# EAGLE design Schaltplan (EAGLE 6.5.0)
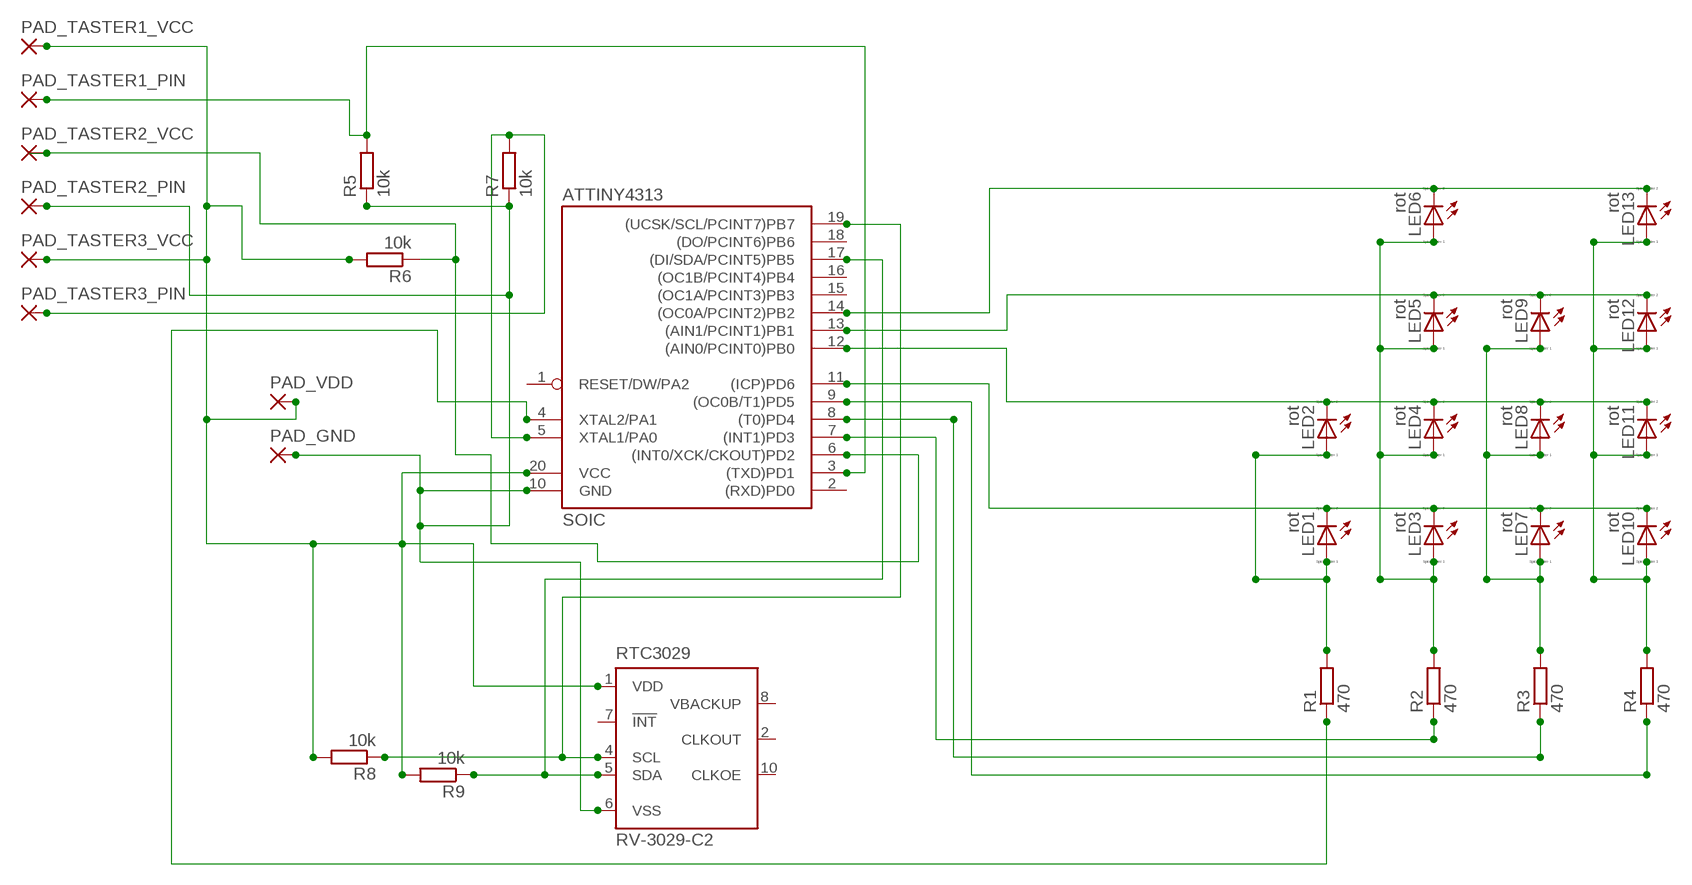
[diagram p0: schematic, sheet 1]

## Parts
ATTINY4313  SOIC  TINY2313P_THM'SOIC'  [SOIC20S]
LED1  rot  LED_ESML0603  [LED_SML0603]
LED2  rot  LED_ESML0603  [LED_SML0603]
LED3  rot  LED_ESML0603  [LED_SML0603]
LED4  rot  LED_ESML0603  [LED_SML0603]
LED5  rot  LED_ESML0603  [LED_SML0603]
LED6  rot  LED_ESML0603  [LED_SML0603]
LED7  rot  LED_ESML0603  [LED_SML0603]
LED8  rot  LED_ESML0603  [LED_SML0603]
LED9  rot  LED_ESML0603  [LED_SML0603]
LED10  rot  LED_ESML0603  [LED_SML0603]
LED11  rot  LED_ESML0603  [LED_SML0603]
LED12  rot  LED_ESML0603  [LED_SML0603]
LED13  rot  LED_ESML0603  [LED_SML0603]
PAD_GND  SMD2  [SMD1,27-2,54]
PAD_TASTER1_PIN  SMD2  [SMD1,27-2,54]
PAD_TASTER1_VCC  SMD2  [SMD1,27-2,54]
PAD_TASTER2_PIN  SMD2  [SMD1,27-2,54]
PAD_TASTER2_VCC  SMD2  [SMD1,27-2,54]
PAD_TASTER3_PIN  SMD2  [SMD1,27-2,54]
PAD_TASTER3_VCC  SMD2  [SMD1,27-2,54]
PAD_VDD  SMD2  [SMD1,27-2,54]
R1  470  R-EU_R0603  [R0603]
R2  470  R-EU_R0603  [R0603]
R3  470  R-EU_R0603  [R0603]
R4  470  R-EU_R0603  [R0603]
R5  10k  R-EU_R0603  [R0603]
R6  10k  R-EU_R0603  [R0603]
R7  10k  R-EU_R0603  [R0603]
R8  10k  R-EU_R0603  [R0603]
R9  10k  R-EU_R0603  [R0603]
RTC3029  RV-3029-C2  [SON-10]

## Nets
N$1: LED1.A LED2.A R1.2
N$2: LED3.A LED4.A LED5.A LED6.A R2.2
N$3: LED7.A LED8.A LED9.A R3.2
N$4: LED10.A LED11.A LED12.A LED13.A R4.2
N$5: ATTINY4313.14((OC0A/PCINT2)PB2) LED6.C LED13.C
N$6: ATTINY4313.13((AIN1/PCINT1)PB1) LED5.C LED9.C LED12.C
N$7: ATTINY4313.12((AIN0/PCINT0)PB0) LED2.C LED4.C LED8.C LED11.C
N$8: ATTINY4313.11((ICP)PD6) LED1.C LED3.C LED7.C LED10.C
N$9: ATTINY4313.9((OC0B/T1)PD5) R4.1
N$10: ATTINY4313.19((UCSK/SCL/PCINT7)PB7) R8.1 RTC3029.4(SCL)
N$11: ATTINY4313.17((DI/SDA/PCINT5)PB5) R9.1 RTC3029.5(SDA)
N$12: ATTINY4313.4(XTAL2/PA1) R1.1
N$13: ATTINY4313.3((TXD)PD1) PAD_TASTER1_PIN.1(P) R5.2
N$14: ATTINY4313.5(XTAL1/PA0) PAD_TASTER3_PIN.1(P) R7.2
N$18: ATTINY4313.8((T0)PD4) R3.1
N$19: ATTINY4313.7((INT1)PD3) R2.1
N$20: ATTINY4313.6((INT0/XCK/CKOUT)PD2) PAD_TASTER2_VCC.1(P) R6.1
N$23: ATTINY4313.20(VCC) PAD_TASTER1_VCC.1(P) PAD_TASTER3_VCC.1(P) PAD_VDD.1(P) R6.2 R8.2 R9.2 RTC3029.1(VDD)
N$24: ATTINY4313.10(GND) PAD_GND.1(P) PAD_TASTER2_PIN.1(P) R5.1 R7.1 RTC3029.6(VSS)
Unconnected: ATTINY4313.1(RESET/DW/PA2) ATTINY4313.2((RXD)PD0) ATTINY4313.15((OC1A/PCINT3)PB3) ATTINY4313.16((OC1B/PCINT4)PB4) ATTINY4313.18((DO/PCINT6)PB6) RTC3029.2(CLKOUT) RTC3029.7(!INT) RTC3029.8(VBACKUP) RTC3029.10(CLKOE)

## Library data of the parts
ATTINY4313 = atmel_THM:TINY2313*P_THM: Features Utilizes the AVR® RISC Architecture AVR® High-performance and Low-power RISC Architecture - 120 Powerful Instructions ? Most Single Clock Cycle Execution - 32 x 8 General Purpose Working Registers - Fully Static Operation Data and Non-volatile Program and Data Memories - 2K Bytes of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
LED1-LED13 = eagle-ltspice:LED_E: LED; SPICEMODEL: NONE; SPICEPREFIX: D; SPICETYPE: diode
PAD_GND PAD_TASTER1_PIN PAD_TASTER1_VCC PAD_TASTER2_PIN PAD_TASTER2_VCC PAD_TASTER3_PIN PAD_TASTER3_VCC PAD_VDD = wirepad:SMD2: SMD PAD
R1-R9 = rcl:R-EU_: RESISTOR, European symbol
RTC3029 = crystal:RV-3029-C2: Highly accurate, DTCXO Temperature Compensated Real Time Clock / Calendar Module with I2C Interface. Source: Data shhet

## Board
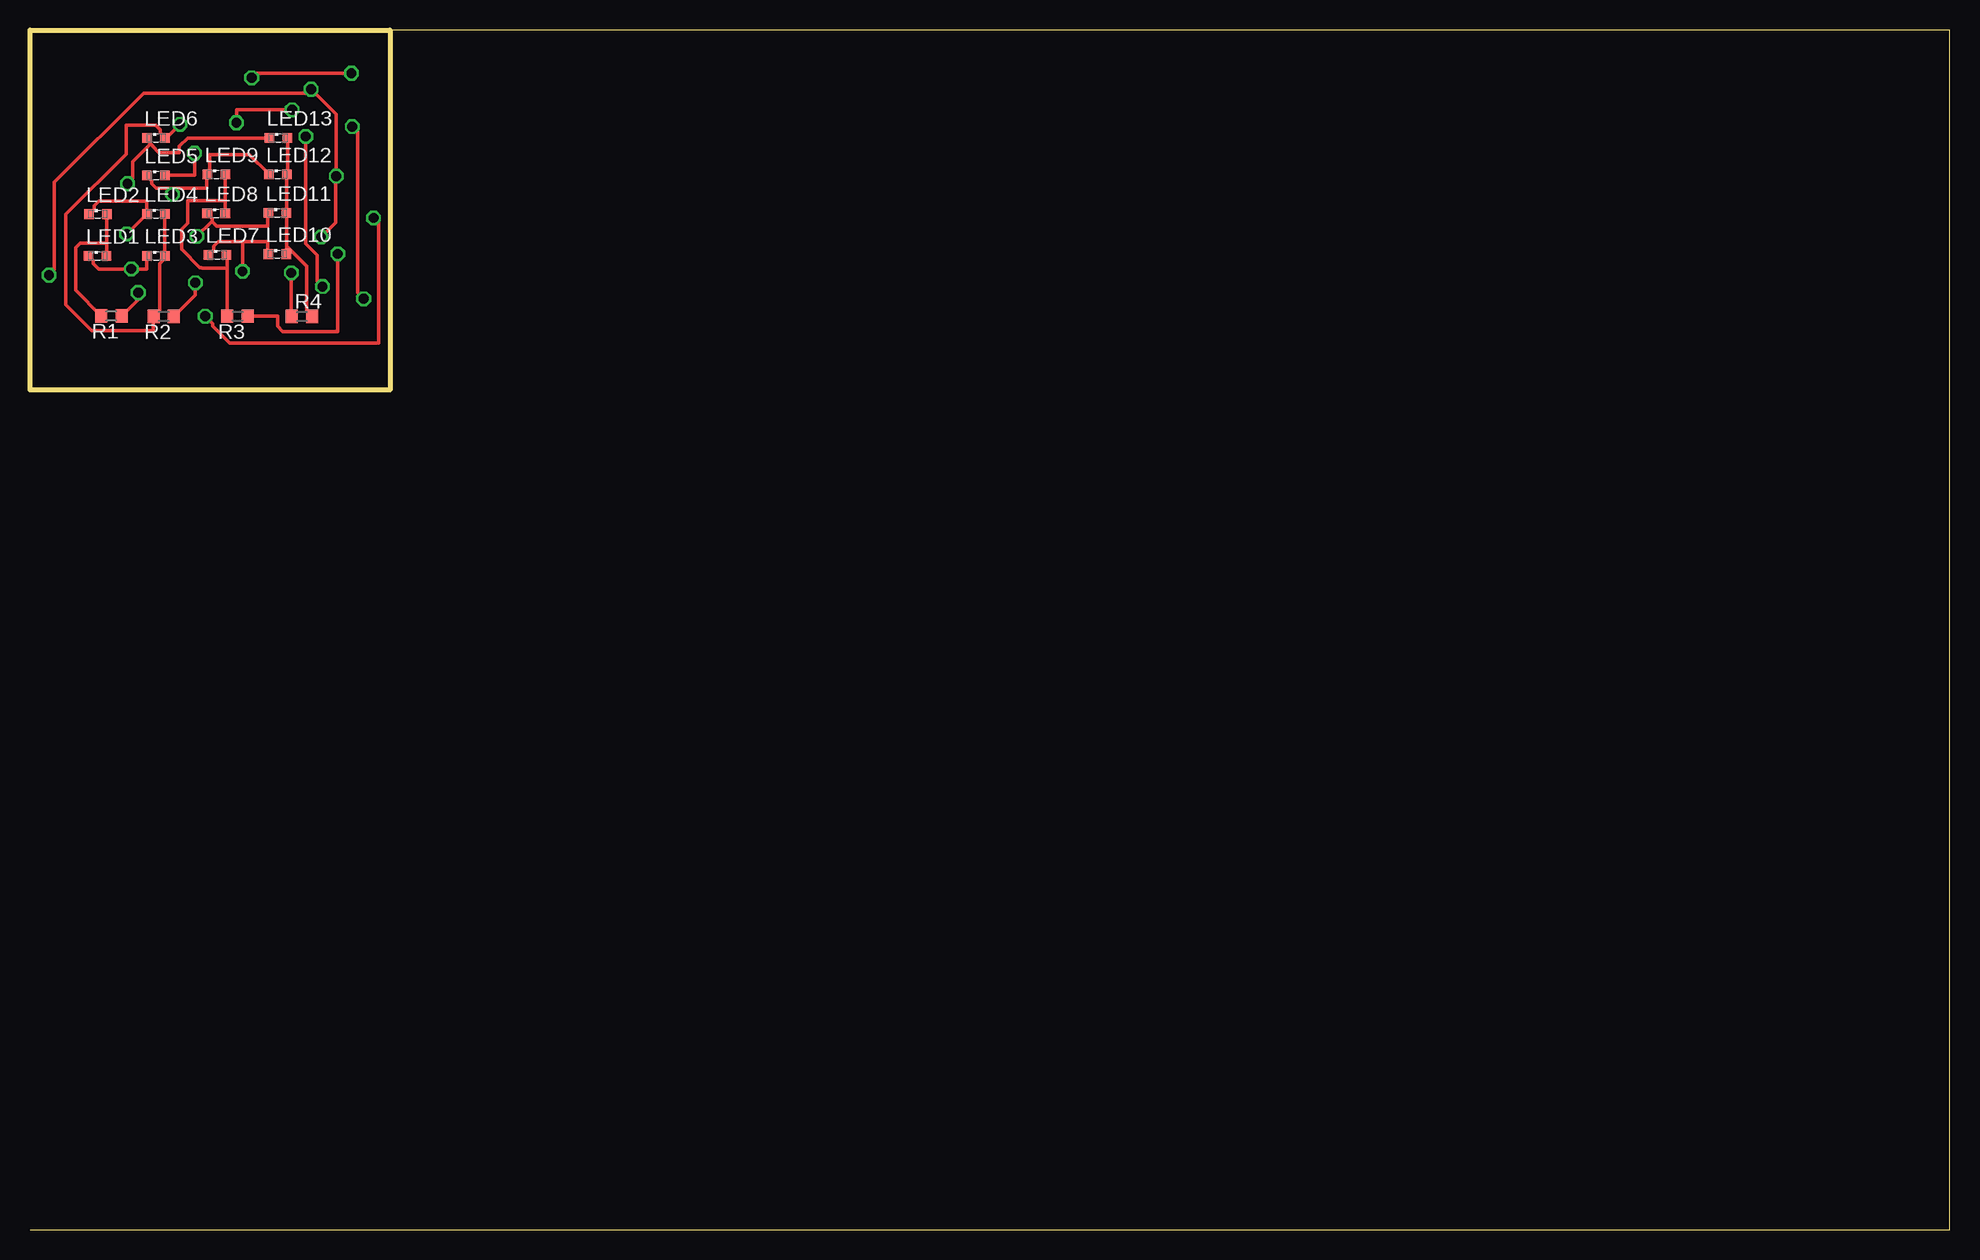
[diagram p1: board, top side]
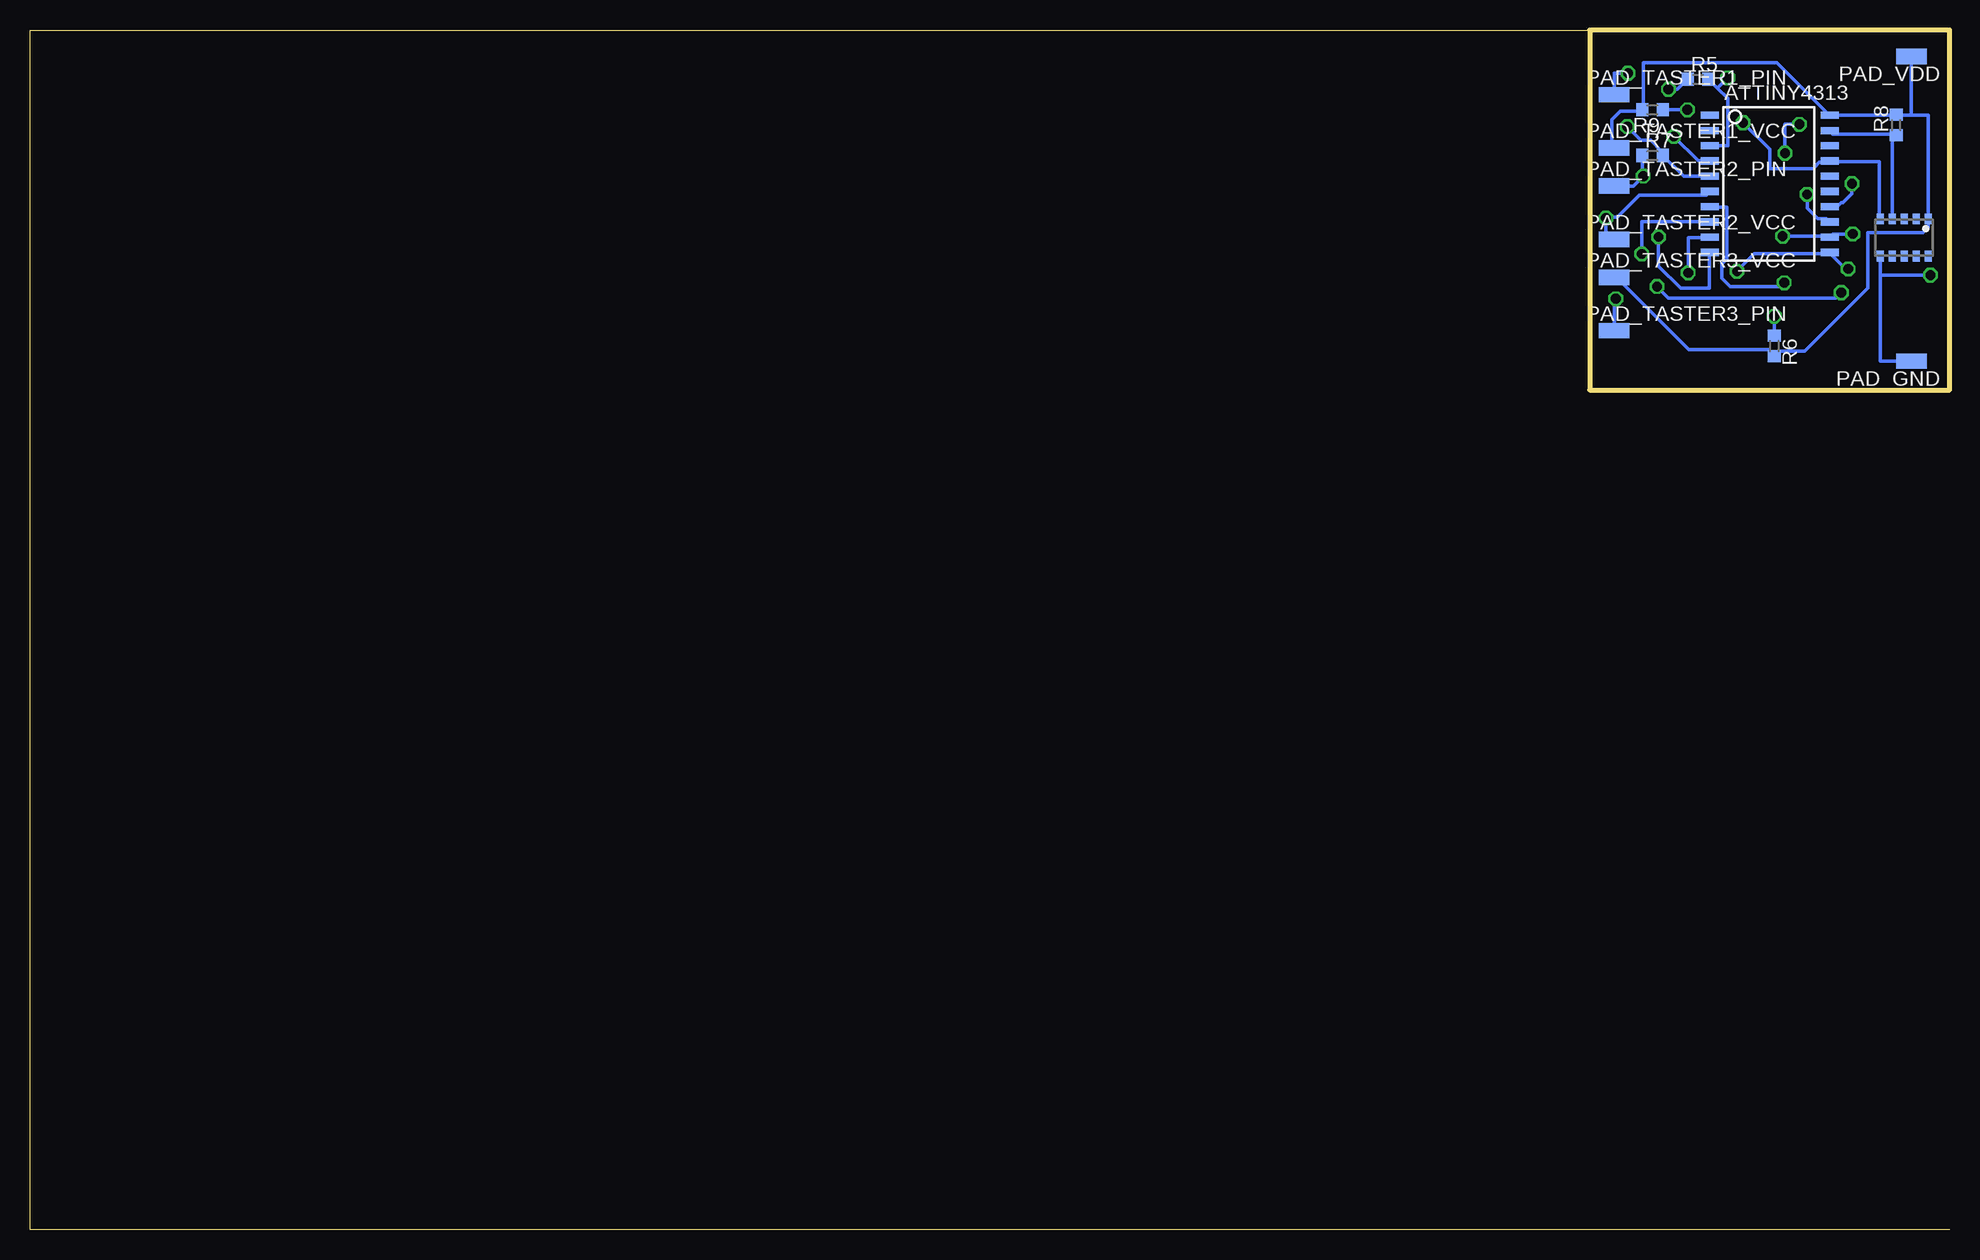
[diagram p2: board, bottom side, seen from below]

Size 160 x 100 mm. Coordinates in mm from the lower left corner, seen from the top.
Outline: 0,0 160,0 160,100 30,100
Outline: 30,100 0,100 0,70 30,70 30,100
Copper layers (1*16): Top 0.035mm / dielectric 1.5mm / Bottom 0.035mm
Design rules "default *": minimum track width 12mil, minimum drill 32mil, track to track 20mil, track to pad 20mil, pad to pad 20mil, via to via 20mil, smd to smd 12mil, copper to edge 20mil, drill to drill 45mil, minimum pad ring 10mil, minimum via ring 8mil, stop-mask expansion 4mil, vias tented up to drill 0mil, thermal gap 10mil
bKeepout: area 1.3,80.6 to 6.3,84.5; area 8.9,80.6 to 21,94

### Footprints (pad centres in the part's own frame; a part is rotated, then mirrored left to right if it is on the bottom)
SOIC20S = smd 0.6 x 1.5: 1 -5.715,-5; 2 -4.445,-5; 3 -3.175,-5; 4 -1.905,-5; 5 -0.635,-5; 6 0.635,-5; 7 1.905,-5; 8 3.175,-5; 9 4.445,-5; 10 5.715,-5; 11 5.715,5; 12 4.445,5; 13 3.175,5; 14 1.905,5; 15 0.635,5; 16 -0.635,5; 17 -1.905,5; 18 -3.175,5; 19 -4.445,5; 20 -5.715,5
LED_SML0603 = smd 0.8 x 0.8: A 0.75,0; C -0.75,0
SMD1,27-2,54 = smd 1.27 x 2.54: 1 0,0
R0603 = smd 1 x 1.1: 1 -0.85,0; 2 0.85,0
SON-10 = smd 0.9 x 0.6: 1 -1.55,2; 2 -1.55,1; 3 -1.55,0; 4 -1.55,-1; 5 -1.55,-2; 6 1.55,-2; 7 1.55,-1; 8 1.55,0; 9 1.55,1; 10 1.55,2

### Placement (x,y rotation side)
ATTINY4313  14.97,87.17 270 bottom
LED1  5.63,81.16 0 top
LED2  5.65,84.64 0 top
LED3  10.52,81.18 0 top
LED4  10.5,84.66 0 top
LED5  10.52,87.87 0 top
LED6  10.5,91 0 top
LED7  15.62,81.25 0 top
LED8  15.52,84.7 0 top
LED9  15.54,87.95 0 top
LED10  20.62,81.31 0 top
LED11  20.61,84.74 0 top
LED12  20.66,87.95 0 top
LED13  20.7,91.01 0 top
PAD_GND  3.17,72.39 90 bottom
PAD_TASTER1_PIN  27.94,94.61 270 bottom
PAD_TASTER1_VCC  27.94,90.17 270 bottom
PAD_TASTER2_PIN  27.94,87 270 bottom
PAD_TASTER2_VCC  27.94,82.55 270 bottom
PAD_TASTER3_PIN  27.94,74.93 270 bottom
PAD_TASTER3_VCC  27.94,79.38 270 bottom
PAD_VDD  3.17,97.79 90 bottom
R1  6.78,76.17 180 top
R2  11.15,76.12 180 top
R3  17.3,76.14 180 top
R4  22.66,76.12 0 top
R5  20.95,95.89 0 bottom
R6  14.61,73.66 270 bottom
R7  24.77,89.53 0 bottom
R8  4.45,92.08 90 bottom
R9  24.77,93.34 180 bottom
RTC3029  3.78,82.7 270 bottom

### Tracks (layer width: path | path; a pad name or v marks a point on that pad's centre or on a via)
N$1
  Top 0.305: 6.41,82.23 6.41,84.58 LED2.A | 6.41,82.23 6.41,81.22 LED1.A | 6.41,82.23 4.19,82.23 3.81,81.85 3.81,78.3 5.91,76.2 R1.2
N$2  (via drill 0.81)
  Top 0.305: LED4.A 11.24,84.64 11.24,81.22 LED3.A 11.3,81.03 10.79,80.52 10.79,76.71 10.35,76.26 R2.2 10.29,76.07 10.29,74.93 5.14,74.93 2.98,77.09 2.98,84.64 8,89.66 8,92.08 10.48,92.08 10.86,91.69 10.86,91.44 11.24,91.06 LED6.A 11.37,91 v12.51,92.14 | v13.72,89.72 13.72,87.88 11.3,87.88 LED5.A
  Bottom 0.305: v13.72,89.72 13.72,92.14 v12.51,92.14
N$3
  Top 0.305: 16.26,85.79 16.26,87.95 LED9.A | 16.26,85.79 16.26,84.71 LED8.A | 16.45,80.14 16.45,76.2 R3.2 | 16.45,80.14 16.45,81.15 16.38,81.22 LED7.A | 16.26,85.79 13.14,85.79 13.14,83.88 12.64,83.38 12.64,81.72 14.16,80.2 14.29,80.2 14.35,80.14 16.45,80.14
N$4
  Top 0.305: 21.4,81.85 21.4,84.64 LED11.A 21.4,84.77 LED12.A 21.46,88.08 21.46,91 LED13.A | 21.4,81.85 21.4,81.34 LED10.A | R4.2 23.5,76.14 23.05,76.58 23.05,80.33 21.53,81.85 21.4,81.85
N$5  (via drill 0.81)
  Top 0.305: 10.03,90.55 10.03,91 9.78,91 LED6.C | 10.03,90.55 10.22,90.36 10.22,90.3 10.73,89.79 12.45,89.79 12.45,90.3 13.14,91 19.94,91 LED13.C | v8.13,87.19 8.57,87.63 8.57,89.03 9.97,90.42 10.03,90.55
  Bottom 0.305: v8.13,87.19 8.13,86.36 8.89,85.6 9.02,85.6 9.34,85.28 9.97,85.28 ATTINY4313.14
N$6  (via drill 0.81)
  Top 0.305: 11.87,86.81 14.73,86.81 14.73,87.95 LED9.C 14.86,88.08 14.99,88.2 14.99,89.6 18.29,89.6 19.88,88.01 LED12.C | 11.87,86.81 10.54,86.81 10.16,87.19 10.16,87.44 9.78,87.82 LED5.C | 11.87,86.81 v11.87,86.3
  Bottom 0.305: v11.87,86.3 11.87,85.15 10.99,84.26 10.29,84.26 10.03,84.01 ATTINY4313.13
N$7  (via drill 0.81)
  Top 0.305: 15.18,84.01 15.18,84.26 14.8,84.64 LED8.C | 15.18,84.01 15.56,83.63 19.81,83.63 19.81,84.71 LED11.C | LED2.C 4.95,84.64 5.33,85.03 5.33,85.34 5.71,85.72 9.72,85.72 9.72,84.71 LED4.C 9.65,84.58 v8.06,83 | v13.91,82.8 15.05,83.95 15.18,84.01
  Bottom 0.305: v8.06,83 9.72,83 ATTINY4313.12 10.1,82.8 v13.91,82.8
N$8  (via drill 0.81)
  Top 0.305: 17.72,82.36 19.81,82.36 19.81,81.34 LED10.C | 17.72,82.36 15.68,82.36 15.3,81.98 15.3,81.66 14.92,81.28 LED7.C | LED1.C 5.27,80.77 5.27,80.52 5.71,80.07 v8.45,80.07 9.72,80.07 9.72,81.15 LED3.C | v17.72,79.88 17.72,82.36
  Bottom 0.305: v8.45,80.07 8.64,80.07 9.97,81.41 ATTINY4313.11 10.1,81.34 16.26,81.34 v17.72,79.88
N$9  (via drill 0.81)
  Top 0.305: v21.78,79.76 21.78,76.14 R4.1
  Bottom 0.305: v21.78,79.76 21.78,82.68 20,82.68 ATTINY4313.9
N$10
  Bottom 0.305: RTC3029.4 4.76,84.26 4.76,91.19 4.45,91.19 R8.1 4.83,91.31 9.72,91.31 9.97,91.57 ATTINY4313.19
N$11  (via drill 0.81)
  Top 0.305: v21.84,93.34 17.21,93.34 v17.21,92.27
  Bottom 0.305: RTC3029.5 5.84,84.26 5.84,89.03 9.97,89.03 ATTINY4313.17 10.1,88.96 10.86,88.96 11.37,88.46 14.99,88.46 14.99,90.04 v17.21,92.27 | v21.84,93.34 R9.1
N$12  (via drill 0.81)
  Top 0.305: v9.02,78.11 9.02,77.53 7.68,76.2 R1.1 | v24.38,78.61 23.94,79.06 23.94,81.22 22.99,82.17 v22.99,91.12
  Bottom 0.305: v9.02,78.11 9.46,77.66 23.43,77.66 v24.38,78.61 | v22.99,91.12 20.95,89.09 20,89.09 ATTINY4313.4
N$13  (via drill 0.81)
  Top 0.305: v26.8,96.39 18.48,96.39 v18.48,96.01
  Bottom 0.305: 19.34,95.16 18.48,94.3 18.48,90.36 19.94,90.36 ATTINY4313.3 | 19.34,95.16 20.07,95.89 R5.2 | PAD_TASTER1_PIN.1 27.94,96.39 v26.8,96.39 | 19.34,95.16 v18.48,96.01
N$14  (via drill 0.81)
  Top 0.305: v27.81,77.6 27.3,78.11 27.3,91.5 v26.86,91.95
  Bottom 0.305: ATTINY4313.5 20,87.82 22.16,87.82 23.88,89.53 R7.2 24,89.66 24,89.92 24.89,90.81 25.72,90.81 v26.86,91.95 | PAD_TASTER3_PIN.1 27.94,77.6 v27.81,77.6
N$18  (via drill 0.81)
  Top 0.305: v25.65,81.34 25.65,74.87 21.08,74.87 20.64,75.31 20.64,76.14 18.16,76.14 R3.1
  Bottom 0.305: v25.65,81.34 25.65,84.01 20,84.01 ATTINY4313.8
N$19  (via drill 0.81)
  Top 0.305: v13.78,78.93 13.78,77.92 12,76.14 R2.1
  Bottom 0.305: v13.78,78.93 14.1,78.61 18.29,78.61 18.99,79.31 18.99,80.52 18.92,80.52 18.54,80.9 18.54,85.22 19.94,85.22 ATTINY4313.7
N$20  (via drill 0.81)
  Top 0.305: v14.61,76.14 15.24,75.5 15.24,75.31 16.64,73.91 29.08,73.91 29.08,83.88 v28.64,84.33
  Bottom 0.305: v14.61,76.14 R6.1 | PAD_TASTER2_VCC.1 28.64,82.55 v28.64,84.33 28.51,84.39 27.69,84.39 25.84,86.23 20.26,86.23 20,86.49 ATTINY4313.6
N$23
  Bottom 0.305: PAD_TASTER3_VCC.1 27.75,79.38 21.72,73.34 15.11,73.34 14.61,72.83 R6.2 14.48,72.9 14.16,73.22 12.06,73.22 6.79,78.49 6.79,83.12 2.22,83.12 1.78,83.57 1.78,84.14 RTC3029.1 1.78,84.26 1.78,92.9 3.17,92.9 | PAD_TASTER1_VCC.1 28.13,90.17 28.13,92.52 27.43,93.22 25.78,93.22 25.65,93.34 R9.2 25.53,93.47 25.53,97.28 14.41,97.28 10.1,92.96 ATTINY4313.20 4.57,92.9 R8.2 4.45,92.9 3.17,92.9 | 3.17,92.9 PAD_VDD.1
N$24  (via drill 0.81)
  Top 0.305: v24.26,82.74 25.46,83.95 25.46,87.69 v25.53,87.82 25.53,92.96 v23.43,95.06 23.3,95 23.3,94.74 9.46,94.74 2.03,87.31 2.03,80.01 v1.59,79.57
  Bottom 0.305: 5.78,79.57 5.78,72.39 PAD_GND.1 | 5.78,79.57 5.78,81.09 RTC3029.6 | v23.43,95.06 22.67,95.06 21.84,95.89 R5.1 | PAD_TASTER2_PIN.1 26.35,87 v25.53,87.82 25.59,87.95 25.59,89.53 R7.1 | v24.26,82.74 24.26,80.33 22.42,78.49 20,78.49 20,81.41 ATTINY4313.10 | v1.59,79.57 5.78,79.57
